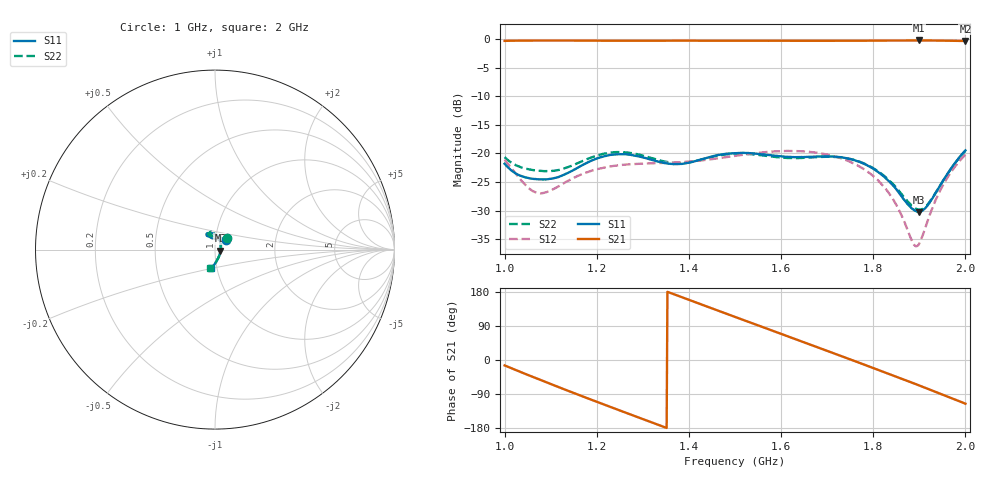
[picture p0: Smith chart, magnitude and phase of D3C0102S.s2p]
! 11/3/2020 4:00:11 PM
! C:\USERS\DITOM\DESKTOP\SINGLE JUNTION ISOLATOR DATA\1.0-2.0 GHZ (D3I0102S).S2P
! CHANNEL.1
! TR.MEASUREMENT
! CORRECTED.DATA
# GHZ S RI R 50.0
! FREQ.GHZ  S11RE  S11IM  S21RE  S21IM  S12RE  S12IM  S22RE  S22IM
!; PortSelection: Port_12
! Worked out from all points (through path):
!   601 points, 1 GHz to 2 GHz, reference 50 ohm
!   highest |S21| = -0.22 dB at 1.9 GHz (marker M1); lowest = -0.3 dB at 2 GHz (marker M2)
!   lowest |S11| = -30.3 dB at 1.9 GHz (marker M3), VSWR 1.06, Z = 53.1 - j0.559 ohm
!   |S11| at or under -10 dB: start of sweep to end of sweep
!   |S22| runs from -29.9 to -19.5 dB; largest |S21 - S12| = 1.1
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1  0.0629 0.0514  0.937 -0.2381  -0.039 0.0791  0.0679 0.0634
1.073333  0.0102 0.0584  0.6183 -0.7513  0.045 0.00118  0.0158 0.0687
1.121667  -0.0127 0.062  0.2736 -0.9343  0.0134 -0.0511  -0.00653 0.0719
1.166667  -0.0302 0.0721  -0.0825 -0.9685  -0.0399 -0.0518  -0.0226 0.0818
1.243333  -0.0323 0.0927  -0.6253 -0.7416  -0.0724 0.0299  -0.0227 0.1001
1.29  -0.0239 0.0913  -0.8507 -0.4645  -0.0327 0.0742  -0.0147 0.0969
1.335  -0.0234 0.0812  -0.9617 -0.1399  0.0269 0.0779  -0.0147 0.086
1.373333  -0.0309 0.0743  -0.9606 0.1556  0.0694 0.0464  -0.0226 0.0788
1.411667  -0.041 0.0745  -0.8684 0.4339  0.0854 -0.00492  -0.0327 0.0789
1.5  -0.0452 0.0898  -0.3913 0.8872  0.00797 -0.0948  -0.0359 0.0922
1.541667  -0.0389 0.0919  -0.0864 0.9647  -0.052 -0.0855  -0.0304 0.0931
1.581667  -0.0345 0.0895  0.2144 0.9454  -0.0936 -0.045  -0.0269 0.0898
1.621667  -0.0331 0.0869  0.4958 0.8326  -0.1045 0.0108  -0.0268 0.0871
1.666667  -0.0315 0.0878  0.7515 0.6106  -0.0787 0.0658  -0.026 0.0885
1.71  -0.0231 0.0911  0.9131 0.3255  -0.0304 0.0908  -0.018 0.0916
1.751667  -0.00716 0.0888  0.9689 0.0141  0.0152 0.0824  -0.00265 0.089
1.793333  0.0113 0.0753  0.9234 -0.3001  0.0408 0.0527  0.0158 0.0753
1.835  0.0265 0.05  0.7764 -0.5868  0.0387 0.0216  0.0297 0.0496
1.886667  0.0317 0.00693  0.4729 -0.8521  0.0121 0.0109  0.0335 0.00653
1.9  0.0302 -0.00526  0.3769 -0.8989  0.00538 0.0154  0.0317 -0.00575
1.948333  0.0155 -0.0528  -0.00303 -0.9714  0.00129 0.0501  0.0151 -0.0527
2  -0.0235 -0.1037  -0.4121 -0.8719  0.0512 0.0828  -0.0253 -0.1024
